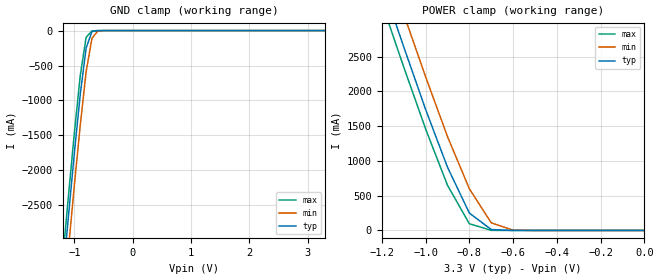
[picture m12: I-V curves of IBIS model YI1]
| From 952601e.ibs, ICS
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|   Model YI1
[Model]   YI1
Model_type   Input
Polarity   Non-Inverting
Enable   Active-High
Vinl =   0.80V
Vinh =   2.00V
C_comp   5.50pF   5.00pF   6.00pF
[Temperature Range]   27.00   70.00   0.000
[Voltage Range]   3.30V   3.00V   3.70V
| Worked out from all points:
|   GND clamp passes 1 mA (typ) near -0.60 V on its own axis
|   POWER clamp passes 1 mA (typ) near -0.61 V on its own axis
[GND_clamp]
| voltage   I(typ)   I(min)   I(max)
-3.3V     -24.05A    -24.49A    -23.79A
-1.2V     -3.55A     -4.02A     -3.26A
-1.1V     -2.63A     -3.1A      -2.34A
-1V       -1.74A     -2.2A      -1.45A
-900mV    -910mA     -1.35A     -640mA
-800mV    -250mA     -590mA     -96.82mA
-700mV    -14.58mA   -110mA     -3.87mA
-600mV    -880uA     -5.82mA    -450uA
-500mV    -88.5uA    -350uA     -45.09uA
3.3V      130pA      250nA      110pA
[POWER_clamp]
| voltage   I(typ)   I(min)   I(max)
-3.3V     24.06A     24.5A      23.8A
-1.2V     3.56A      4.03A      3.27A
-1.1V     2.64A      3.11A      2.35A
-1V       1.74A      2.21A      1.46A
-900mV    910mA      1.35A      650mA
-800mV    250mA      600mA      96.92mA
-700mV    13.09mA    110mA      2.11mA
-600mV    300uA      5.19mA     34.41uA
0V        130pA      310pA      130pA
